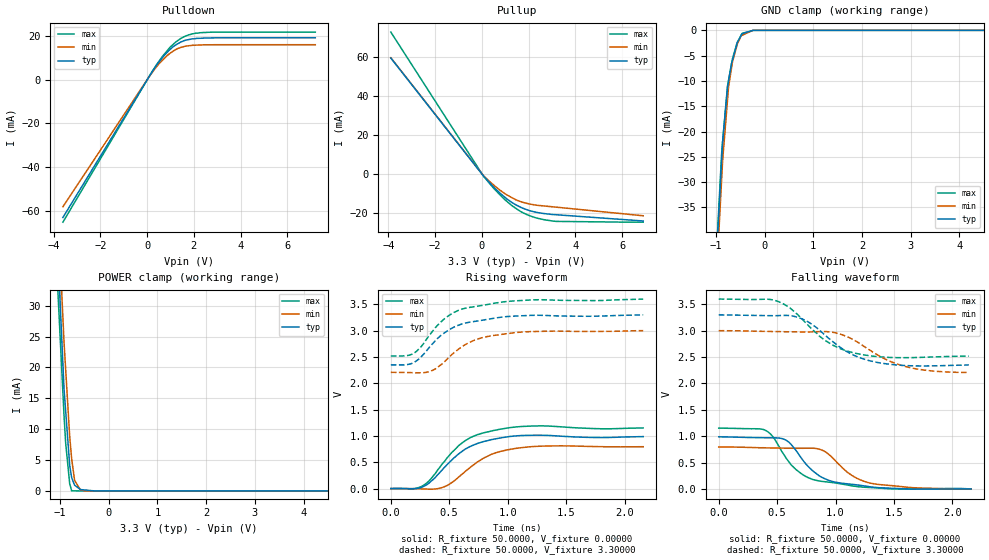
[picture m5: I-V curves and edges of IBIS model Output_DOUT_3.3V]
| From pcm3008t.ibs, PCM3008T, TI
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[Model] Output_DOUT_3.3V
Model_type Output
Vref  = 0.00000V
Cref  = 2.00000pF
Vmeas = 1.65000V
C_comp  1.57000pF 1.57000pF 1.57000pF
[Model spec]
|   typ   min   max
Vmeas  1.6500V  1.5000V  1.8000V
| variable   typ   min   max
[Voltage Range]   3.30000V  3.00000V  3.60000V
[POWER Clamp Reference]  3.30000V  3.00000V  3.60000V
[Pullup Reference]   3.30000V  3.00000V  3.60000V
[Pulldown Reference]   0.00000V  0.00000V  0.00000V
[GND Clamp Reference]   0.00000V  0.00000V  0.00000V
[Temperature Range]   25   85   -25
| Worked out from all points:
|   slope of the pulldown table from 0 to 0.495 V, typ, clamps not added: 61.8 ohm
|   slope of the pullup table from 0 to 0.495 V, typ, clamps not added: 74.8 ohm
|   GND clamp passes 1 mA (typ) near -0.48 V on its own axis
|   POWER clamp passes 1 mA (typ) near -0.70 V on its own axis
|   rising waveform, R_fixture 50.0000, V_fixture 0.00000: 20-80 % time 296ps typ, 298ps min, 286ps max; typ from 0 V to 0.988 V
|   falling waveform, R_fixture 50.0000, V_fixture 0.00000: 20-80 % time 263ps typ, 275ps min, 265ps max; typ from 0.988 V to 0 V
|   falling waveform, R_fixture 50.0000, V_fixture 3.30000: 20-80 % time 347ps typ, 388ps min, 335ps max; typ from 3.3 V to 2.35 V
|   rising waveform, R_fixture 50.0000, V_fixture 3.30000: 20-80 % time 312ps typ, 307ps min, 303ps max; typ from 2.35 V to 3.3 V
[GND Clamp]
-3.6V     -518.5mA   -526.3mA   -529.8mA
-3V       -409.7mA   -416.7mA   -418.3mA
-881.1mV  -25.6mA    -29.44mA   -24.28mA
-861.2mV  -21.99mA   -25.8mA    -22.09mA
-760mV    -11.24mA   -13.7mA    -10.96mA
-739.7mV  -10.08mA   -11.28mA   -9.897mA
-679.1mV  -6.618mA   -7.504mA   -6.702mA
-658.9mV  -5.905mA   -6.247mA   -5.638mA
-562.2mV  -2.498mA   -2.793mA   -2.419mA
-461.7mV  -652.8uA   -994.3uA   -607.9uA
-240.8mV  -28.29uA   0A         -26.32uA
7.2V      0A         0A         0A
[Pulldown]
-3.6V     -63.09mA   -58.17mA   -65.24mA
81.27mV   1.266mA    1.239mA    1.273mA
522mV     8.219mA    7.405mA    8.592mA
739.7mV   11.13mA    9.744mA    11.69mA
982.5mV   13.81mA    12.06mA    14.83mA
1.219V    15.84mA    13.75mA    17.15mA
1.639V    18.03mA    15.31mA    19.93mA
1.942V    18.7mA     15.73mA    21.01mA
2.261V    18.95mA    15.89mA    21.51mA
7.2V      19.18mA    16.01mA    21.79mA
[Pullup]
-3.9V     59.25mA    59.4mA     72.55mA
77.7mV    -1.381mA   -1.187mA   -1.445mA
497.8mV   -6.852mA   -5.781mA   -7.427mA
761.3mV   -9.881mA   -8.351mA   -10.7mA
1.281V    -14.75mA   -12.29mA   -16.38mA
1.661V    -17.26mA   -14.34mA   -19.44mA
2.081V    -19.11mA   -15.64mA   -21.71mA
2.621V    -20.39mA   -16.5mA    -23.5mA
3.041V    -20.93mA   -17mA      -24.28mA
6.9V      -24.24mA   -21.57mA   -24.86mA
[POWER Clamp]
-3.9V     536.8mA    530.4mA    488.5mA
-1.079V   44.74mA    51.55mA    38mA
-917.8mV  16.57mA    24.13mA    12.21mA
-884.5mV  13mA       19.75mA    7.807mA
-801.7mV  4.147mA    8.853mA    1.185mA
-761.3mV  2.155mA    5.216mA    21.09uA
-700.4mV  931.3uA    1.694mA    13.83uA
-579mV    221.2uA    148.9uA    0A
-477.9mV  144uA      0A         0A
-289.5mV  0A         0A         0A
6.9V      0A         0A         0A
[Rising Waveform]
R_fixture = 50.0000
V_fixture = 0.00000
V_fixture_min = 0.00000
V_fixture_max = 0.00000
0s        0V         0V         0V
200ps     -2.711mV   -2mV       998uV
280ps     40.37mV    -6.727mV   62.28mV
440ps     357.3mV    20.56mV    468.5mV
580ps     657.9mV    218.1mV    815.2mV
680ps     801.5mV    402.9mV    967.8mV
800ps     896.5mV    586.1mV    1.063V
940ps     963mV      707.4mV    1.13V
1.2ns     1.013V     796mV      1.188V
2.16ns    987.8mV    795.7mV    1.153V
[Falling Waveform]
R_fixture = 50.0000
V_fixture = 0.00000
V_fixture_min = 0.00000
V_fixture_max = 0.00000
0s        987.8mV    795.7mV    1.153V
400ps     969.1mV    778.1mV    1.11V
460ps     968.5mV    775.6mV    999mV
580ps     917.6mV    771.7mV    573mV
700ps     606.4mV    770mV      299.1mV
820ps     314.9mV    769.6mV    169.1mV
980ps     136.2mV    574.1mV    117.5mV
1.14ns    86.24mV    254.3mV    57.38mV
1.28ns    44.72mV    118.7mV    27.3mV
2.16ns    0V         0V         0V
[Falling Waveform]
R_fixture = 50.0000
V_fixture = 3.30000
V_fixture_min = 3.00000
V_fixture_max = 3.60000
0s        3.3V       3V         3.6V
460ps     3.285V     2.985V     3.586V
560ps     3.29V      2.981V     3.501V
680ps     3.251V     2.977V     3.296V
780ps     3.147V     2.977V     3.068V
920ps     2.897V     2.983V     2.803V
1.18ns    2.512V     2.795V     2.567V
1.4ns     2.382V     2.49V      2.502V
1.58ns    2.341V     2.331V     2.488V
2.14ns    2.35V      2.208V     2.518V
[Rising Waveform]
R_fixture = 50.0000
V_fixture = 3.30000
V_fixture_min = 3.00000
V_fixture_max = 3.60000
0s        2.35V      2.208V     2.518V
140ps     2.355V     2.205V     2.527V
200ps     2.397V     2.201V     2.574V
260ps     2.503V     2.2V       2.697V
340ps     2.711V     2.23V      2.939V
480ps     2.99V      2.455V     3.261V
640ps     3.145V     2.737V     3.428V
800ps     3.204V     2.877V     3.487V
1.12ns    3.283V     2.973V     3.573V
2.16ns    3.3V       3V         3.6V
[Ramp]
| variable typ min max
dV/dt_r 590.605m/326.348p 475.853m/326.268p 688.573m/307.716p
dV/dt_f 572.578m/347.202p 476.454m/388.409p 649.867m/335.384p
R_load = 50.0000Ohms
